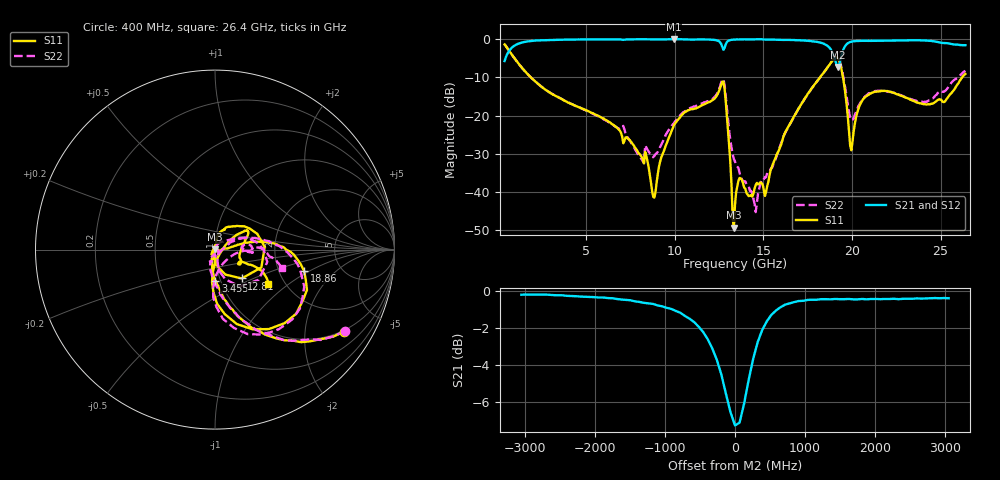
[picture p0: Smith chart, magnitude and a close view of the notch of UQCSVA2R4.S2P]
!  Part Number  UQCSVA2R4  Mounting Orientation: Horizontal
!  Description: Ultra Low ESR Microwave capacitors
!  Application: Coupling, Bypass, Tuning, DC Block
!  Filters, Matching
# GHZ S DB R 50
! Freq  |S11|  S11 Ph  |S21|  S21 Ph  |S12|  S12 Ph  |S22|  S22 Ph
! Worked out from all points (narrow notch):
!   401 points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, 400 MHz to 26.4 GHz, reference 50 ohm
!   highest |S21| = 0.01 dB at 9.955 GHz (marker M1); lowest = -7.3 dB at 19.18 GHz (marker M2)
!   notch at M2: 7.0 dB deep, 512 MHz wide at half that depth
!   lowest |S11| = -49.3 dB at 13.34 GHz (marker M3), VSWR 1.01, Z = 49.7 + j0.228 ohm
!   |S11| at or under -10 dB: 1.876 GHz to 18.2 GHz (16.32 GHz wide, 163 % of centre); 19.49 GHz to 26.21 GHz (6.721 GHz wide, 29.4 % of centre)
!   |S22| runs from -45.3 to -1.4 dB; largest |S21 - S12| = 0.0099
!   S11 on the Smith chart (normalised r, x): 400 MHz: 0.95, -3.19; 3.455 GHz: 0.95, -0.34; 12.81 GHz: 1.27, -0.43; 18.86 GHz: 2.76, -0.89; 26.4 GHz: 1.64, -0.71
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0.4  -1.38 -32.4  -5.74 57.4  -5.74 57.3  -1.36 -32.1
1.375  -7.48 -68.6  -0.89 20.5  -0.87 20.6  -7.48 -68.8
3.455  -15.26 -89.3  -0.17 -2.2  -0.17 -2.3  -15.24 -92.0
4.755  -18.10 -95.5  -0.09 -10.0  -0.10 -10.1  -18.20 -101.2
7.55  -26.97 -98.0  -0.05 -23.4  -0.05 -23.5  -27.21 -114.1
8.785  -41.27 164.4  -0.07 -29.3  -0.06 -29.3  -30.91 -41.2
9.11  -33.38 91.0  -0.08 -30.6  -0.07 -30.6  -28.83 -7.1
9.955  -22.54 79.3  0.01 -34.6  0.01 -34.7  -22.01 21.6
12.815  -13.18 -47.2  -2.24 -39.1  -2.21 -39.6  -12.08 -55.9
13.335  -49.34 137.7  -0.12 -45.8  -0.13 -45.8  -31.37 -45.9
13.4  -43.33 96.0  -0.11 -46.4  -0.12 -46.4  -32.03 -37.0
13.66  -36.34 74.1  -0.08 -48.5  -0.08 -48.5  -35.05 -17.4
14.57  -38.18 -6.1  -0.04 -53.7  -0.06 -53.9  -45.27 63.8
15.155  -39.88 -37.1  -0.11 -57.2  -0.11 -57.2  -36.16 77.3
17.755  -12.70 11.1  -0.57 -73.2  -0.55 -73.3  -12.74 16.4
18.86  -5.83 -13.5  -3.12 -88.8  -3.12 -88.8  -5.83 -18.1
19.185  -4.97 -46.5  -7.29 -71.6  -7.22 -71.7  -4.90 -51.2
19.965  -29.08 -22.1  -0.68 -61.0  -0.66 -61.0  -21.23 -52.2
20.615  -15.80 33.6  -0.44 -71.0  -0.45 -70.9  -15.64 -2.1
22.11  -13.74 25.5  -0.40 -82.5  -0.40 -82.5  -13.81 -3.9
24.45  -16.94 -15.9  -0.46 -101.2  -0.49 -101.2  -15.87 8.3
26.4  -9.10 -32.8  -1.59 -115.6  -1.58 -115.4  -8.29 -15.8
